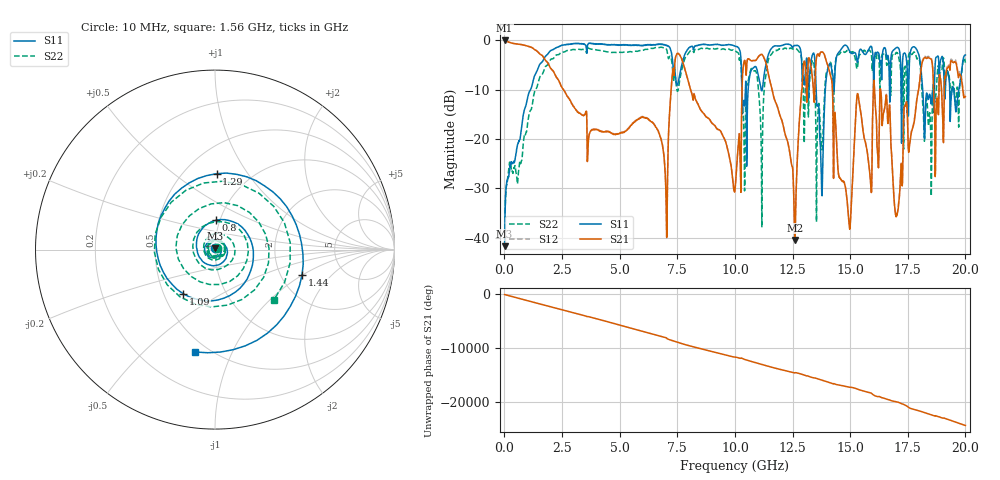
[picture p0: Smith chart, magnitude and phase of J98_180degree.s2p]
!Keysight Technologies,N5222A,MY51421036,A.10.65.16
!Date: Friday, March 31, 2023 14:40:28
!Correction: S11(Full 2 Port(1,2))
!S21(Full 2 Port(1,2))
!S12(Full 2 Port(1,2))
!S22(Full 2 Port(1,2))
!S2P File: Measurements: S11, S21, S12, S22:
# Hz S  dB  R 50
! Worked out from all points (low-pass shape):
!   2000 points, 10 MHz to 20 GHz, reference 50 ohm
!   highest |S21| = -0.05 dB at 10 MHz (marker M1); lowest = -40.4 dB at 12.6 GHz (marker M2)
!   |S21| within 3 dB of the highest: start of sweep to 1.63 GHz; 13.68 GHz to 13.89 GHz (214.6 MHz wide, 1.56 % of centre)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
!   lowest |S11| = -41.7 dB at 10 MHz (marker M3), VSWR 1.02, Z = 50 + j0.822 ohm
!   |S11| at or under -10 dB: start of sweep to 1.136 GHz; 13.52 GHz to 13.92 GHz (399.9 MHz wide, 2.91 % of centre); 18.15 GHz to 18.65 GHz (504.2 MHz wide, 2.74 % of centre)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
!   |S22| runs from -38.3 to -1.4 dB; largest |S21 - S12| = 0.036
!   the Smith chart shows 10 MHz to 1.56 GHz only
!   S11 on the Smith chart (normalised r, x): 10 MHz: 1.00, +0.02; 800 MHz: 0.96, +0.32; 1.09 GHz: 0.63, -0.34; 1.29 GHz: 0.71, +0.73; 1.44 GHz: 2.61, -0.99; 1.56 GHz: 0.42, -0.73
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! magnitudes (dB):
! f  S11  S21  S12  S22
! 10 MHz  -41.7  -0.1  0.0  -38.3
! 800 MHz  -15.7  -0.9  -0.9  -21.9
! 1.09 GHz  -10.4  -1.3  -1.3  -14.6
! 1.29 GHz  -7.5  -1.8  -1.8  -10.8
! 1.44 GHz  -5.9  -2.3  -2.3  -9.1
! 1.56 GHz  -4.7  -2.8  -2.8  -7.3
! 3.35 GHz  -0.7  -15.0  -15.0  -1.9
! 6.68 GHz  -0.8  -18.5  -18.4  -1.5
! 7.01 GHz  -1.1  -31.3  -31.2  -1.6
! 7.57 GHz  -7.9  -2.8  -2.7  -9.2
! 10.01 GHz  -1.2  -30.1  -30.0  -2.1
! 10.42 GHz  -13.3  -4.1  -4.1  -30.5
! 11.15 GHz  -10.1  -2.9  -2.8  -25.0
! 12.6 GHz  -1.1  -40.4  -40.3  -1.8
! 13.34 GHz  -3.4  -6.6  -6.5  -4.6
! 13.77 GHz  -31.3  -2.4  -2.4  -22.0
! 14.96 GHz  -2.0  -37.5  -37.5  -2.3
! 15.33 GHz  -4.3  -10.8  -10.7  -5.1
! 16.67 GHz  -4.1  -15.2  -15.0  -4.1
! 17.02 GHz  -1.5  -35.2  -35.4  -2.5
! 18.2 GHz  -15.5  -3.7  -3.4  -17.9
! 20 GHz  -3.0  -11.4  -10.9  -4.6
